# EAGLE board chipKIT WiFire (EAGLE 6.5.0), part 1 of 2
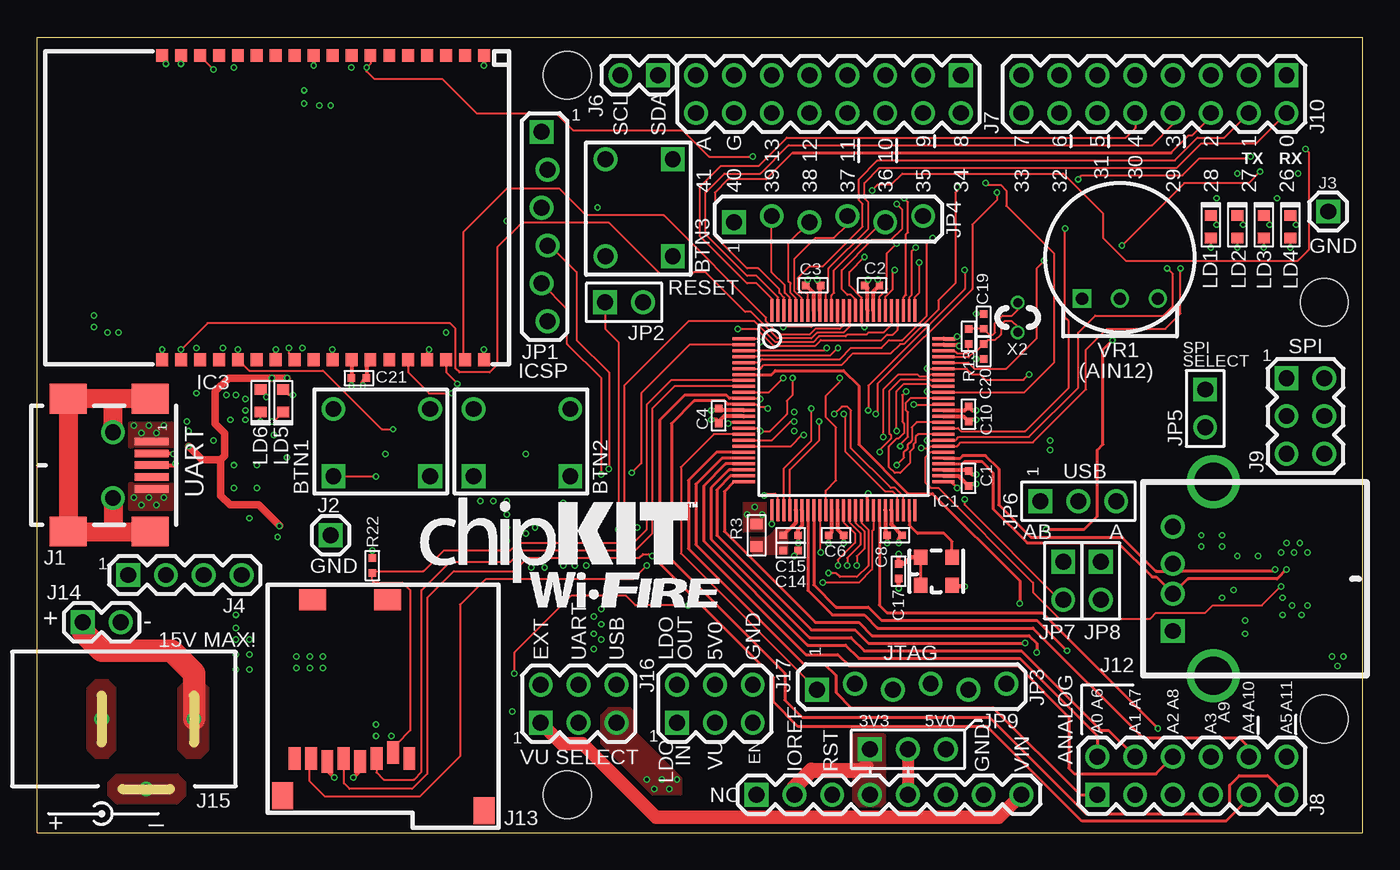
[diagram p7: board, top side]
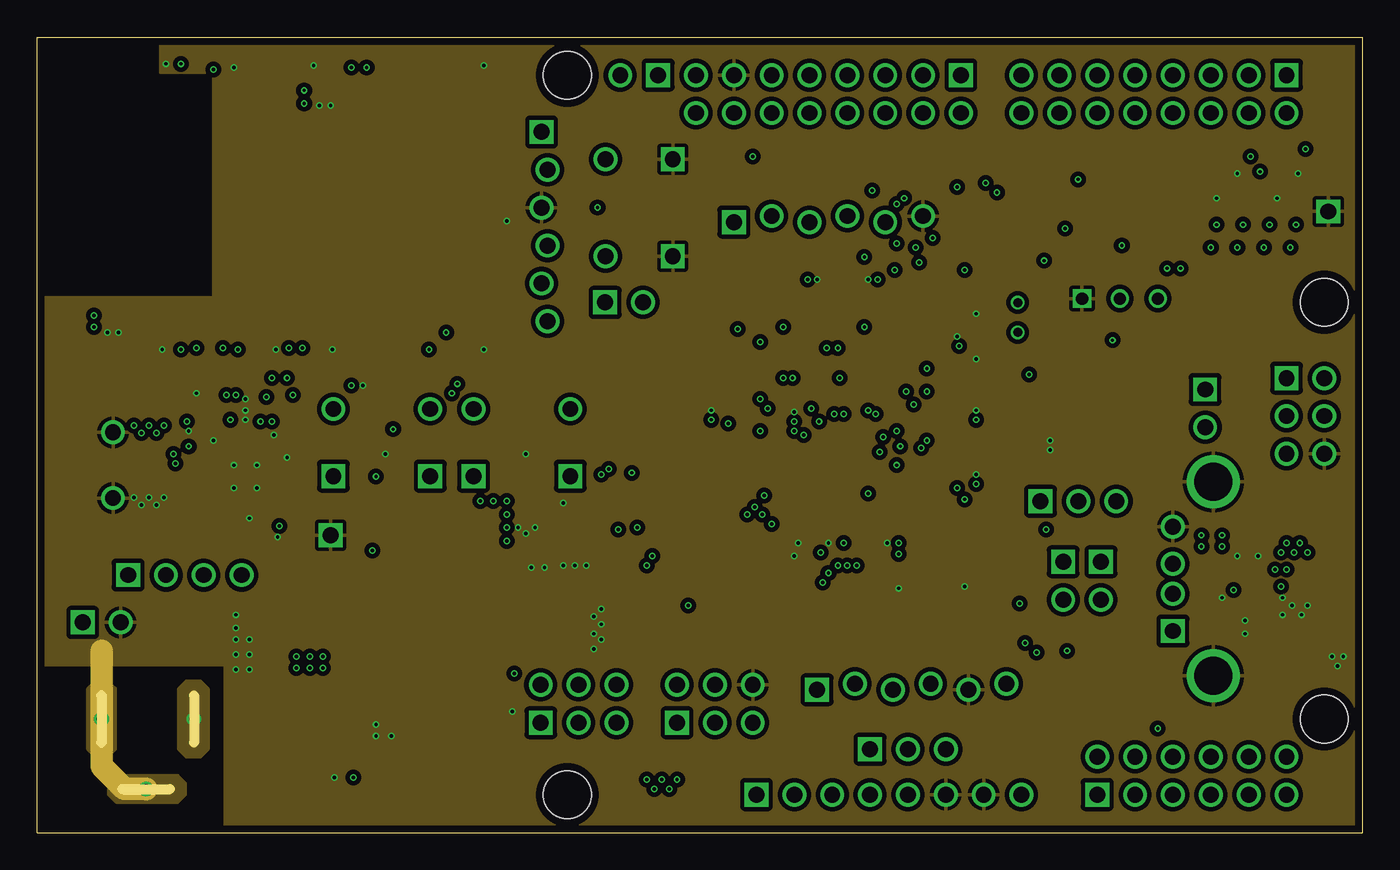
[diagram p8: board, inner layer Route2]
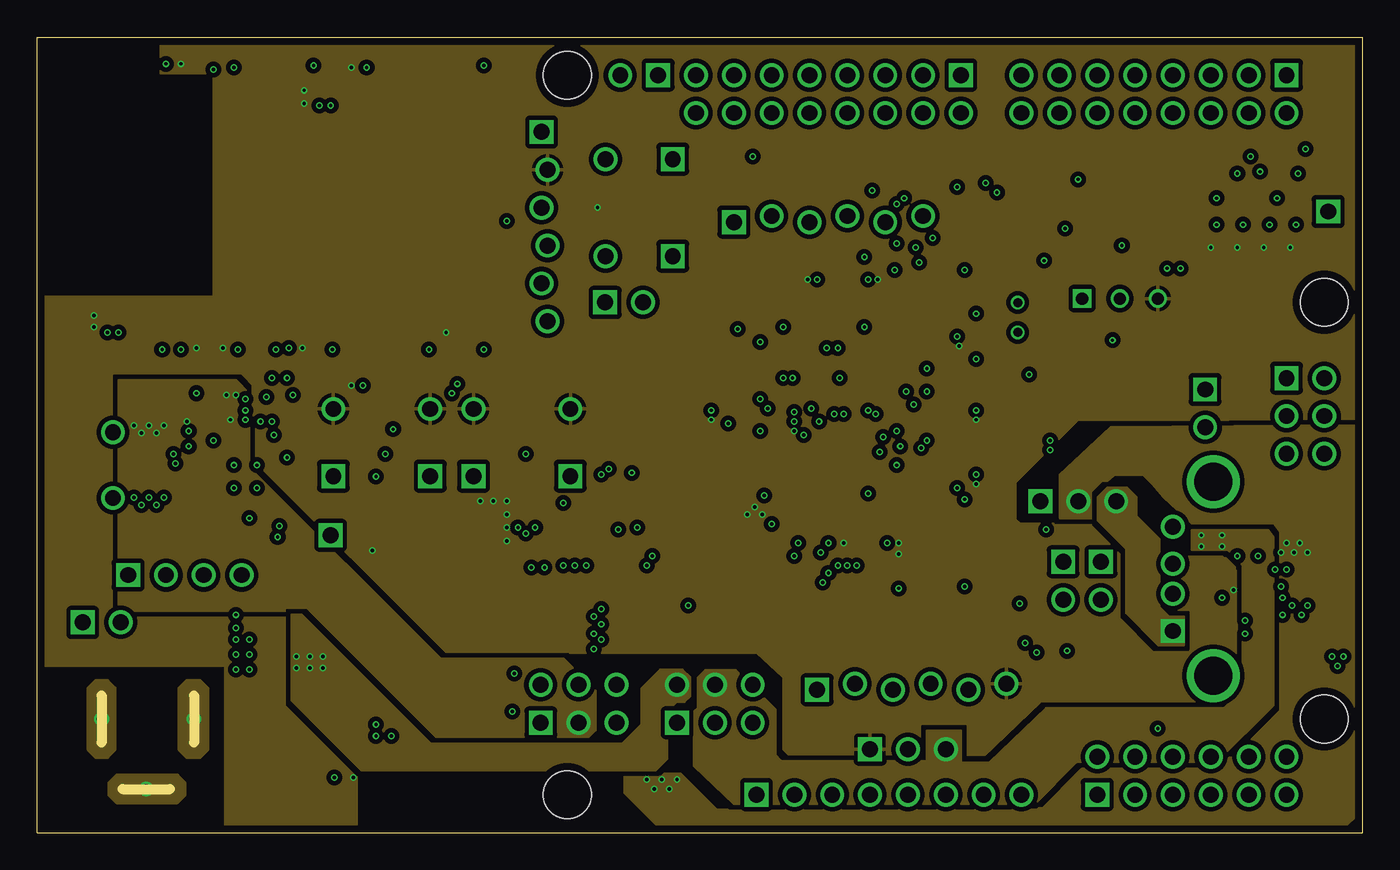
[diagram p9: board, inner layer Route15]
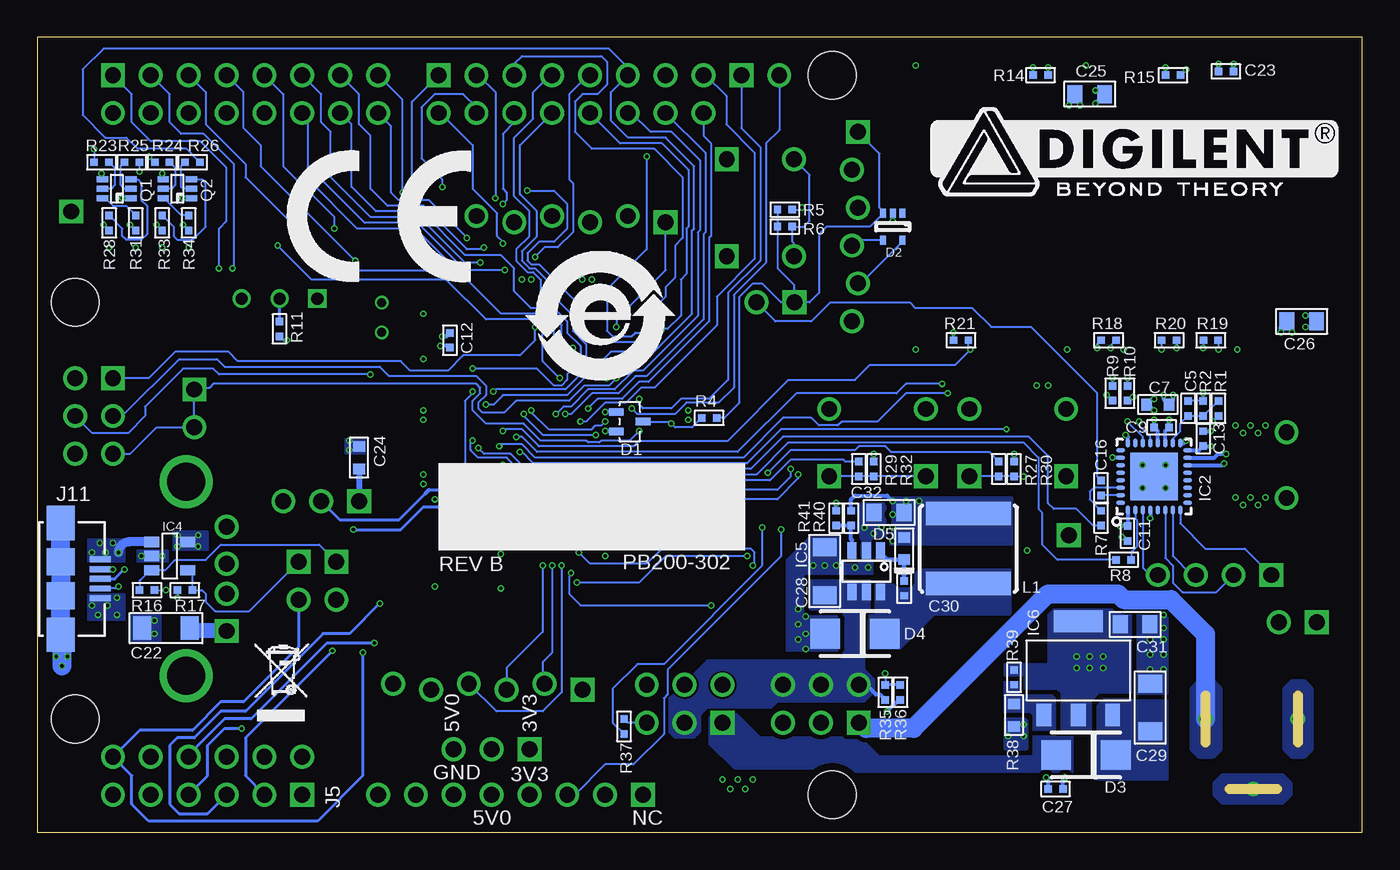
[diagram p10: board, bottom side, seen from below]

Size 88.9 x 53.34 mm. Coordinates in mm from the lower left corner, seen from the top.
Outline: 0,0 0,53.34 88.9,53.34 88.9,0 0,0
Copper layers ((1*2)+(15*16)): Top 0.035mm / dielectric 0.4mm / Route2 0.035mm / dielectric 0.66mm / Route15 0.035mm / dielectric 0.4mm / Bottom 0.035mm
Design rules "default *": minimum track width 5mil, minimum drill 9mil, track to track 5mil, track to pad 5mil, pad to pad 5mil, via to via 5mil, smd to smd 5mil, copper to edge 20mil, drill to drill 8mil, minimum pad ring 2mil, minimum via ring 2mil, stop-mask expansion 4mil, vias tented up to drill 15mil, thermal gap 10mil
Holes 3.2 mm at 35.56,50.8 86.36,35.56 86.36,7.62 35.56,2.54

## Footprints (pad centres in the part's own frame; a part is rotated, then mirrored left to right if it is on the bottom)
SW-P8008 = drill 1.067 square: 1A -2,3.5; 2A -2,-3 | drill 1.067: 1B 2.5,3.5; 2B 2.5,-3
C0402S = smd 0.5 x 0.5: 1 -0.5,0; 2 0.5,0
C0603S = smd 0.7 x 0.8: 1 -0.75,0; 2 0.75,0
C1206S = smd 1.2 x 1.6: 1 -1.6,0; 2 1.6,0
C0805S = smd 1 x 1.2: 1 -1,0; 2 1,0
SOT-323 = smd 0.5 x 1: 1 -0.65,-0.9; 2 0.65,-0.9; 3 0,0.9
SOT-323-5 = smd 0.4 x 0.6: 1 -0.65,-0.9; 2 0,-0.9; 3 0.65,-0.9; 4 0.65,0.9; 5 -0.65,0.9
SMA = smd 2 x 2: A 2,0; C -2,0
D0603S = smd 0.7 x 0.8: A 0.75,0; C -0.75,0
TQ100-PT = smd 1.5 x 0.2: 1 -6.7,4.8; 2 -6.7,4.4; 3 -6.7,4; 4 -6.7,3.6; 5 -6.7,3.2; 6 -6.7,2.8; 7 -6.7,2.4; 8 -6.7,2; 9 -6.7,1.6; 10 -6.7,1.2; 11 -6.7,0.8; 12 -6.7,0.4; 13 -6.7,0; 14 -6.7,-0.4; 15 -6.7,-0.8; 16 -6.7,-1.2; 17 -6.7,-1.6; 18 -6.7,-2; 19 -6.7,-2.4; 20 -6.7,-2.8; 21 -6.7,-3.2; 22 -6.7,-3.6; 23 -6.7,-4; 24 -6.7,-4.4; 25 -6.7,-4.8; 51 6.7,-4.8; 52 6.7,-4.4; 53 6.7,-4; 54 6.7,-3.6; 55 6.7,-3.2; 56 6.7,-2.8; 57 6.7,-2.4; 58 6.7,-2; 59 6.7,-1.6; 60 6.7,-1.2; 61 6.7,-0.8; 62 6.7,-0.4; 63 6.7,0; 64 6.7,0.4; 65 6.7,0.8; 66 6.7,1.2; 67 6.7,1.6; 68 6.7,2; 69 6.7,2.4; 70 6.7,2.8; 71 6.7,3.2; 72 6.7,3.6; 73 6.7,4; 74 6.7,4.4; 75 6.7,4.8 | smd 0.2 x 1.5: 26 -4.8,-6.7; 27 -4.4,-6.7; 28 -4,-6.7; 29 -3.6,-6.7; 30 -3.2,-6.7; 31 -2.8,-6.7; 32 -2.4,-6.7; 33 -2,-6.7; 34 -1.6,-6.7; 35 -1.2,-6.7; 36 -0.8,-6.7; 37 -0.4,-6.7; 38 0,-6.7; 39 0.4,-6.7; 40 0.8,-6.7; 41 1.2,-6.7; 42 1.6,-6.7; 43 2,-6.7; 44 2.4,-6.7; 45 2.8,-6.7; 46 3.2,-6.7; 47 3.6,-6.7; 48 4,-6.7; 49 4.4,-6.7; 50 4.8,-6.7; 76 4.8,6.7; 77 4.4,6.7; 78 4,6.7; 79 3.6,6.7; 80 3.2,6.7; 81 2.8,6.7; 82 2.4,6.7; 83 2,6.7; 84 1.6,6.7; 85 1.2,6.7; 86 0.8,6.7; 87 0.4,6.7; 88 0,6.7; 89 -0.4,6.7; 90 -0.8,6.7; 91 -1.2,6.7; 92 -1.6,6.7; 93 -2,6.7; 94 -2.4,6.7; 95 -2.8,6.7; 96 -3.2,6.7; 97 -3.6,6.7; 98 -4,6.7; 99 -4.4,6.7; 100 -4.8,6.7
QFN32 = smd 0.6 x 0.3: 1 -2.25,1.75; 2 -2.25,1.25; 3 -2.25,0.75; 4 -2.25,0.25; 5 -2.25,-0.25; 6 -2.25,-0.75; 7 -2.25,-1.25; 8 -2.25,-1.75; 17 2.25,-1.75; 18 2.25,-1.25; 19 2.25,-0.75; 20 2.25,-0.25; 21 2.25,0.25; 22 2.25,0.75; 23 2.25,1.25; 24 2.25,1.75 | smd 0.3 x 0.6: 9 -1.75,-2.25; 10 -1.25,-2.25; 11 -0.75,-2.25; 12 -0.25,-2.25; 13 0.25,-2.25; 14 0.75,-2.25; 15 1.25,-2.25; 16 1.75,-2.25; 25 1.75,2.25; 26 1.25,2.25; 27 0.75,2.25; 28 0.25,2.25; 29 -0.25,2.25; 30 -0.75,2.25; 31 -1.25,2.25; 32 -1.75,2.25 | smd 3.2 x 3.2: PAD 0,0
MRF24WB0MA = smd 0.85 x 0.8: 1 -10.2,11.43; 2 -10.2,10.16; 3 -10.2,8.89; 4 -10.2,7.62; 5 -10.2,6.35; 6 -10.2,5.08; 7 -10.2,3.81; 8 -10.2,2.54; 9 -10.2,1.27; 10 -10.2,0; 11 -10.2,-1.27; 12 -10.2,-2.54; 13 -10.2,-3.81; 14 -10.2,-5.08; 15 -10.2,-6.35; 16 -10.2,-7.62; 17 -10.2,-8.89; 18 -10.2,-10.16; 19 10.2,-10.16; 20 10.2,-8.89; 21 10.2,-7.62; 22 10.2,-6.35; 23 10.2,-5.08; 24 10.2,-3.81; 25 10.2,-2.54; 26 10.2,-1.27; 27 10.2,0; 28 10.2,1.27; 29 10.2,2.54; 30 10.2,3.81; 31 10.2,5.08; 32 10.2,6.35; 33 10.2,7.62; 34 10.2,8.89; 35 10.2,10.16; 36 10.2,11.43
SOT23-5 = smd 0.7 x 1: 1 -0.95,-1.2; 2 0,-1.2; 3 0.95,-1.2; 4 0.95,1.2; 5 -0.95,1.2
SOT23-6-CH = smd 0.6 x 1.1: 1 -0.95,-1.4; 2 0,-1.4; 3 0.95,-1.4; 4 0.95,1.4; 5 0,1.4; 6 -0.95,1.4
SOT223 = smd 1 x 1.5: 1 -2.3,0; 2 0,0; 3 2.3,0 | smd 3.3 x 1.5: TAB 0,6.3
DSC1033-C = smd 0.9 x 1: 1 -1.05,-0.95; 2 1.05,-0.95; 3 1.05,0.95; 4 -1.05,0.95
USB-AB-MINI = smd 0.5 x 2.3: 1 -1.6,2.6; 2 -0.8,2.6; 3 0,2.6; 4 0.8,2.6; 5 1.6,2.6 | smd 2 x 2.5: S1 -4.45,2.5; S2 -4.45,-3; S3 4.45,-3; S4 4.45,2.5 | drill 1.067: S5 -2.2,0; S6 2.2,0
HDR-1X1 = drill 1.067 square: 1 0,0
HDR-1X4 = drill 1.067 square: 1 0,3.81 | drill 1.067: 2 0,1.27; 3 0,-1.27; 4 0,-3.81
HDR-1X8 = drill 1.067 square: 1 0,8.89 | drill 1.067: 2 0,6.35; 3 0,3.81; 4 0,1.27; 5 0,-1.27; 6 0,-3.81; 7 0,-6.35; 8 0,-8.89
HDR-1X2 = drill 1.067 square: 1 0,1.27 | drill 1.067: 2 0,-1.27
HDR-2X8 = drill 1.067 square: 1 -1.27,8.89 | drill 1.067: 2 1.27,8.89; 3 -1.27,6.35; 4 1.27,6.35; 5 -1.27,3.81; 6 1.27,3.81; 7 -1.27,1.27; 8 1.27,1.27; 9 -1.27,-1.27; 10 1.27,-1.27; 11 -1.27,-3.81; 12 1.27,-3.81; 13 -1.27,-6.35; 14 1.27,-6.35; 15 -1.27,-8.89; 16 1.27,-8.89
HDR-2X6 = drill 1.067 square: 1 -1.27,6.35 | drill 1.067: 2 1.27,6.35; 3 -1.27,3.81; 4 1.27,3.81; 5 -1.27,1.27; 6 1.27,1.27; 7 -1.27,-1.27; 8 1.27,-1.27; 9 -1.27,-3.81; 10 1.27,-3.81; 11 -1.27,-6.35; 12 1.27,-6.35
HDR-2X3 = drill 1.067 square: 1 -1.27,2.54 | drill 1.067: 2 1.27,2.54; 3 -1.27,0; 4 1.27,0; 5 -1.27,-2.54; 6 1.27,-2.54
USB-AB-MICRO = smd 0.4 x 1.4: 1 -1.3,4.1; 2 -0.65,4.1; 3 0,4.1; 4 0.65,4.1; 5 1.3,4.1 | smd 1.8 x 1.9: S1 -1.15,1.45; S2 1.14,1.45 | smd 2.3 x 1.9: S3 -3.75,1.45; S4 3.75,1.45
USB-A = drill 1.067 square: 1 -3.5,0 | drill 1.067: 2 -1,0; 3 1,0; 4 3.5,0 | drill 2.54: S1 -6.5,-2.71; S2 6.5,-2.71
2908-05WB-MG = smd 0.8 x 1.5: 1 -1.6,4.05; 2 -0.5,3.65; 3 0.6,4.05; 4 1.7,4.25; 5 2.8,4.05; 6 3.9,4.25; 7 5,4.05; 8 6.1,4.05 | smd 1.8 x 1.4: P$9 4.9,-6.6; P$10 -0.15,-6.6 | smd 1.4 x 1.8: P$11 -6.6,7.55; P$12 6.9,6.55
KLD-0202S = drill 0.66: 1 6.2,0; 2 0,0; 3 3,-4.7
HDR-1X6_OFFSET = drill 1.067 square: 1 -0.203,6.35 | drill 1.067: 2 0.203,3.81; 3 -0.203,1.27; 4 0.203,-1.27; 5 -0.203,-3.81; 6 0.203,-6.35
JPR-1X2 = drill 1.067 square: 1 0,1.27 | drill 1.067: 2 0,-1.27
JPR-1X3 = drill 1.067 square: 1 0,2.54 | drill 1.067: 2 0,0; 3 0,-2.54
NR60XX = smd 1.6 x 5.7: 1 -2.35,0; 2 2.35,0
SOT-363 = smd 0.4 x 0.762: 1 -0.635,-0.953; 2 0,-0.953; 3 0.635,-0.953; 4 0.635,0.953; 5 0,0.953; 6 -0.635,0.953
R0402S = smd 0.5 x 0.5: 1 -0.5,0; 2 0.5,0
R0603S = smd 0.7 x 0.8: 1 -0.75,0; 2 0.75,0
BOURNS-3352T = drill 0.813 square: 1 -2.54,0 | drill 0.813: 2 0,0; 3 2.54,0
XT-T38 = drill 0.61: 1 -1,0; 2 1,0

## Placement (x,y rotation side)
BTN1  SW-P8008  [SW-P8008]  23.37,25.91 90 top
BTN2  SW-P8008  [SW-P8008]  32.77,25.91 90 top
BTN3  SW-P8008  [SW-P8008]  40.64,42.16 180 top
C1  0.1uF  [C0402S]  62.48,23.75 90 top
C2  0.1uF  [C0402S]  56.01,36.7 180 top
C3  0.1uF  [C0402S]  52.07,36.7 0 top
C4  0.1uF  [C0402S]  45.72,27.94 90 top
C5  0.1uF  [C0402S]  11.68,28.45 90 bottom
C6  0.1uF  [C0402S]  53.59,19.94 180 top
C7  4.7uF  [C0603S]  13.72,28.7 180 bottom
C8  0.1uF  [C0402S]  57.53,19.94 180 top
C9  0.1uF  [C0402S]  13.46,27.18 180 bottom
C10  0.1uF  [C0402S]  62.48,28.07 90 top
C11  0.1uF  [C0402S]  15.75,20.07 270 bottom
C12  0.1uF  [C0402S]  61.21,33.02 90 bottom
C13  0.1uF  [C0402S]  10.67,26.42 90 bottom
C14  1uF  [C0402S]  50.55,18.92 0 top
C15  0.1uF  [C0402S]  50.55,19.94 0 top
C16  0.1uF  [C0402S]  17.53,23.11 90 bottom
C17  0.1uF  [C0402S]  57.78,17.53 270 top
C19  27pF  [C0402S]  63.5,34.29 90 top
C20  20pF  [C0402S]  63.5,32.26 270 top
C21  0.1uF  [C0402S]  21.59,30.48 0 top
C22  100uF/10V  [C1206S]  80.26,13.72 180 bottom
C23  0.1uF  [C0402S]  9.14,51.05 0 bottom
C24  6.8uF/10V  [C0603S]  67.31,25.15 90 bottom
C25  10uF  [C0805S]  18.29,49.53 180 bottom
C26  10uF  [C0805S]  4.06,34.29 180 bottom
C27  0.1uF  [C0402S]  20.57,2.92 0 bottom
C28  10uF/35V  [C1206S]  36.07,17.53 90 bottom
C29  10uF/35V  [C1206S]  14.22,8.38 90 bottom
C30  100nF  [C0402S]  30.73,16.38 270 bottom
C31  10uF/10V  [C0805S]  15.24,13.97 0 bottom
C32  10uF  [C0805S]  31.75,21.46 180 bottom
D1  BAV99W  [SOT-323]  49.15,27.56 270 bottom
D2  NSQA6V8  [SOT-323-5]  31.5,40.64 180 bottom
D3  B240A-13-F  [SMA]  18.54,5.21 180 bottom
D4  B240A-13-F  [SMA]  34.04,13.34 180 bottom
D5  CDSU4148  [D0603S]  30.73,19.05 90 bottom
IC1  PIC32MZ2048ECG100-PT  [TQ100-PT]  54.1,28.32 0 top
IC2  FT232RQ  [QFN32]  13.97,23.88 90 bottom
IC3  MRF24WG0MA  [MRF24WB0MA]  18.54,41.91 270 top
IC4  TPS2051BDBVR  [SOT23-5]  80.01,18.54 270 bottom
IC5  MCP16301T-I/CHY  [SOT23-6-CH]  33.27,17.53 180 bottom
IC6  NCP1117DT50T3G  [SOT223]  19.05,7.87 0 bottom
IC7  DSC1033-CC2-024.000  [DSC1033-C]  60.33,17.53 0 top
J1  KMAB-SMT-5S  [USB-AB-MINI]  5.08,24.64 270 top
J2  ST. Male  [HDR-1X1]  19.68,19.94 0 top
J3  ST. Male  [HDR-1X1]  86.61,41.66 90 top
J4  No Load  [HDR-1X4]  9.91,17.27 90 top
J5  ST. Female  [HDR-1X8]  57.15,2.54 90 top
J6  ST. Female  [HDR-1X2]  40.39,50.8 270 top
J7  ST. Female  [HDR-2X8]  53.09,49.53 270 top
J8  ST. Female  [HDR-2X6]  77.47,3.81 90 top
J9  ST. Male  [HDR-2X3]  85.09,27.94 0 top
J10  ST. Female  [HDR-2X8]  74.93,49.53 270 top
J11  UMMCF-051MBCB-CF535  [USB-AB-MICRO]  88.77,17.02 270 bottom
J12  KUSB-AS-1  [USB-A]  76.2,17.02 90 top
J13  2908-05WB-MG  [2908-05WB-MG]  23.37,9.02 180 top
J14  ST. Male  [HDR-1X2]  4.32,14.1 90 top
J15  CON-COAX-KLD0202-S  [KLD-0202S]  4.32,7.62 0 top
J16  ST. Male  [HDR-2X3]  36.32,8.64 90 top
J17  ST. Male  [HDR-2X3]  45.47,8.64 90 top
JP1  No Load  [HDR-1X6_OFFSET]  34.04,40.64 0 top
JP2  ST. Male  [JPR-1X2]  39.37,35.56 90 top
JP3  No Load  [HDR-1X6_OFFSET]  58.67,9.78 90 top
JP4  No Load  [HDR-1X6_OFFSET]  53.09,41.15 90 top
JP5  No Load  [JPR-1X2]  78.36,28.45 0 top
JP6  ST. Male  [JPR-1X3]  69.85,22.23 90 top
JP7  ST. Male  [JPR-1X2]  68.83,16.89 0 top
JP8  ST. Male  [JPR-1X2]  71.37,16.89 0 top
JP9  JPR-1X3  [JPR-1X3]  58.42,5.59 90 top
L1  NR6028T150M  [NR60XX]  26.42,19.05 90 bottom
LD1  Green  [D0603S]  78.74,40.64 270 top
LD2  Green  [D0603S]  80.52,40.64 270 top
LD3  Green  [D0603S]  82.3,40.64 270 top
LD4  Green  [D0603S]  84.07,40.64 270 top
LD5  Red  [D0603S]  16.51,28.96 90 top
LD6  Red  [D0603S]  14.99,28.96 90 top
LOGO1  DIGILENT_INC-BT-1000  [DIGILENT_BEYOND_1000_LOGO]  28.96,42.67 0 bottom
LOGO2  CE  [CE_LOGO]  72.39,36.83 0 bottom
LOGO3  WEEE-S  [WEEE_LOGO]  73.79,6.73 0 bottom
LOGO4  ROHS-CHINA  [ROHS_CHINA_LOGO]  57.15,29.59 0 bottom
Q1  MBT3904DW1T1  [SOT-363]  83.57,43.18 90 bottom
Q2  MBT3904DW1T1  [SOT-363]  79.5,43.18 90 bottom
R1  4.7K  [R0402S]  9.65,28.45 270 bottom
R2  10K  [R0402S]  10.67,28.45 270 bottom
R3  0  [R0603S]  48.26,19.94 270 top
R4  50  [R0402S]  43.81,27.81 0 bottom
R5  10K  [R0402S]  38.73,41.78 0 bottom
R6  200  [R0402S]  38.73,40.64 180 bottom
R7  1K  [R0402S]  17.53,21.08 270 bottom
R8  1K  [R0402S]  16,18.29 180 bottom
R9  470  [R0402S]  16.76,29.46 90 bottom
R10  470  [R0402S]  15.75,29.46 90 bottom
R11  1K  [R0402S]  72.64,33.78 90 bottom
R13  0  [R0402S]  62.48,33.27 270 top
R14  10K  [R0402S]  21.59,50.8 0 bottom
R15  10K  [R0402S]  12.7,50.8 0 bottom
R16  10K  [R0402S]  81.53,16.26 0 bottom
R17  10K  [R0402S]  78.99,16.26 0 bottom
R18  4.7K  [R0402S]  17.02,33.02 180 bottom
R19  10K  [R0402S]  10.16,33.02 180 bottom
R20  10K  [R0402S]  12.95,33.02 0 bottom
R21  10K  [R0402S]  26.92,33.02 180 bottom
R22  10K  [R0402S]  22.48,17.91 90 top
R23  4.7K  [R0402S]  84.58,44.96 0 bottom
R24  4.7K  [R0402S]  80.52,44.96 0 bottom
R25  4.7K  [R0402S]  82.55,44.96 180 bottom
R26  4.7K  [R0402S]  78.49,44.96 180 bottom
R27  10K  [R0402S]  24.38,24.38 270 bottom
R28  470  [R0402S]  84.07,40.89 270 bottom
R29  10K  [R0402S]  33.78,24.38 270 bottom
R30  10K  [R0402S]  23.37,24.38 270 bottom
R31  470  [R0402S]  82.3,40.89 270 bottom
R32  10K  [R0402S]  32.77,24.38 270 bottom
R33  470  [R0402S]  80.52,40.89 270 bottom
R34  470  [R0402S]  78.74,40.89 270 bottom
R35  10K  [R0402S]  32,9.4 270 bottom
R36  1K  [R0402S]  30.99,9.4 90 bottom
R37  1K  [R0402S]  49.53,7.11 90 bottom
R38  0  [R0603S]  23.37,7.87 90 bottom
R39  NL  [R0402S]  23.37,10.41 90 bottom
R40  31.2K/1%  [R0402S]  34.29,21.08 90 bottom
R41  10K/1%  [R0402S]  35.31,21.08 270 bottom
U$1  CHIPKIT_WIFIRE_LOGO  [CHIPKIT_WIFIRE_LOGO]  25.65,15.11 0 top
VR1  10K  [BOURNS-3352T]  72.64,35.81 0 top
X2  No Load  [XT-T38]  65.79,34.54 270 top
